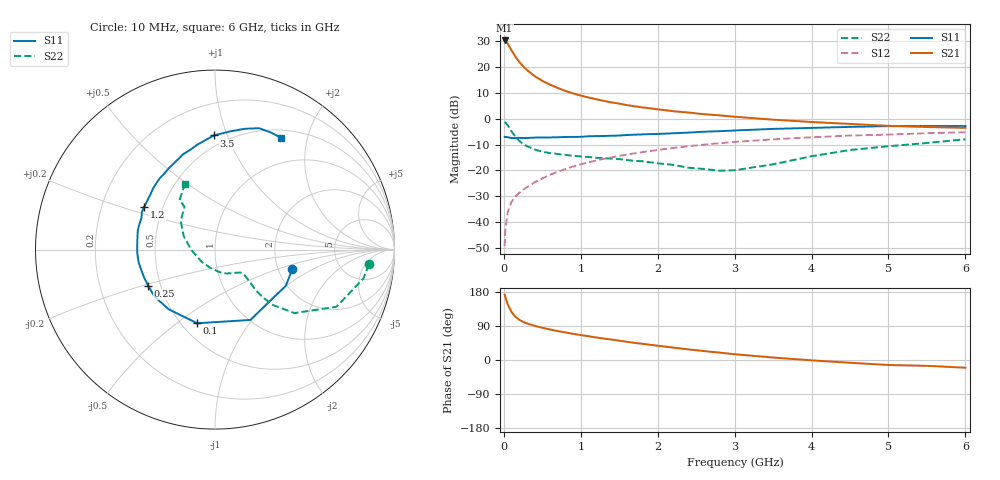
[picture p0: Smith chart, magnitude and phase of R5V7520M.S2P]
! SIEMENS Small Signal Semiconductors
! BFR183
! Si NPN RF Bipolar Junction Transistor in SOT23
! VCE = 0.75 V  IC = 20 mA
! Common Emitter S-Parameters:  May  1996
# GHz  S  MA  R  50
!  f  S11  S21  S12  S22
! GHz  MAG  ANG  MAG  ANG  MAG  ANG  MAG  ANG
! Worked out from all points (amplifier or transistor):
!   36 points, 10 MHz to 6 GHz, reference 50 ohm
!   highest |S21| = 30.3 dB at 10 MHz (marker M1)
!   |S21| within 3 dB of that: start of sweep to 84.05 MHz
!   unconditionally stable (mu >= 1): 323.6 MHz to 4.125 GHz; 5.66 GHz to end of sweep
!   at 250 MHz: K = 0.92, MSG = 23.9 dB, |S12| = -27.5 dB
!   at 1.4 GHz: K = 1.14, MAG = 8.4 dB, |S12| = -15.0 dB
!   at 6 GHz: K = 1.01, MAG = 0.3 dB, |S12| = -5.2 dB
!   S11 on the Smith chart (normalised r, x): 10 MHz: 2.39, -0.65; 100 MHz: 0.60, -0.60; 250 MHz: 0.43, -0.21; 1.2 GHz: 0.39, +0.24; 3.5 GHz: 0.42, +0.90; 6 GHz: 0.61, +1.58
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0.01  0.4449 -14.1  32.84 172.8  0.0034 78.8  0.862 -5.5
0.02  0.4431 -27.1  32.31 165.5  0.0069 79.5  0.8418 -11.1
0.05  0.4386 -63.3  28.51 147.1  0.0155 69.8  0.7479 -25.2
0.1  0.4222 -103.6  21.13 126.7  0.0246 61.3  0.5669 -38.6
0.15  0.4209 -127.7  15.95 114.0  0.0311 60.2  0.4495 -43.6
0.2  0.4269 -141.8  12.63 106.2  0.0367 60.8  0.3729 -45.0
0.25  0.4234 -151.5  10.39 100.7  0.042 61.5  0.3234 -44.9
0.3  0.4246 -159.1  8.798 96.5  0.0473 63.6  0.2948 -44.1
0.4  0.4312 -170.1  6.71 90.2  0.0588 65.4  0.254 -42.5
0.5  0.4338 -177.4  5.406 84.9  0.07 66.5  0.2291 -41.3
0.6  0.4342 176.1  4.573 80.5  0.082 67.0  0.2164 -40.8
0.8  0.4432 166.0  3.462 72.7  0.1059 66.5  0.1995 -41.4
0.9  0.4443 161.3  3.092 69.1  0.1187 66.0  0.1912 -42.0
1.1  0.4576 153.0  2.578 62.7  0.1428 64.4  0.1814 -45.6
1.2  0.461 149.0  2.39 59.6  0.155 63.6  0.1754 -47.1
1.7  0.491 132.7  1.738 45.2  0.2139 57.7  0.1525 -59.0
2.2  0.5225 119.1  1.4 32.8  0.2713 51.1  0.1279 -78.9
2.8  0.5735 103.8  1.164 19.6  0.3357 42.3  0.0985 -120.5
3.5  0.636 90.6  0.959 6.5  0.3984 31.6  0.1308 -178.4
4.5  0.6949 75.8  0.793 -7.3  0.4719 17.6  0.2481 140.4
5.5  0.723 64.3  0.691 -15.4  0.5253 6.1  0.3393 125.6
6  0.7236 59.4  0.667 -20.4  0.5471 -1.3  0.4002 114.9
